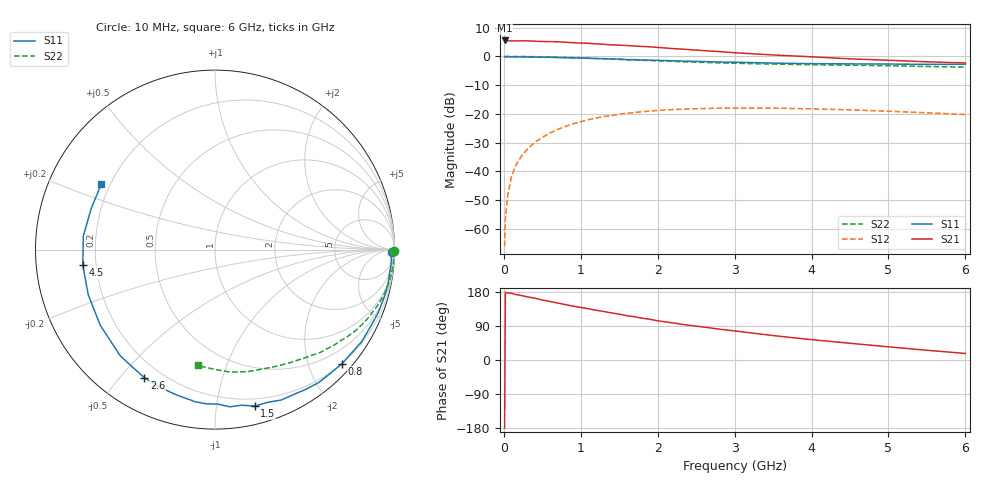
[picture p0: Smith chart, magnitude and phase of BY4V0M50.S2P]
! SIEMENS Small Signal Semiconductors
! BFY420
! Si NPN RF SIEGET Grounded Emitter Transistor in MICRO-X
! VCE = 4 V  IC = 0.5 mA
! Common Emitter S-Parameters:  October  1996
# GHz  S  MA  R  50
!  f  S11  S21  S12  S22
! GHz  MAG  ANG  MAG  ANG  MAG  ANG  MAG  ANG
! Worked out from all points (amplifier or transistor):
!   36 points, 10 MHz to 6 GHz, reference 50 ohm
!   highest |S21| = 5.6 dB at 10 MHz (marker M1)
!   |S21| within 3 dB of that: start of sweep to 2.304 GHz
!   unconditionally stable (mu >= 1): 4.699 GHz to end of sweep
!   at 250 MHz: K = 0.04, MSG = 19.7 dB, |S12| = -34.0 dB
!   at 1.4 GHz: K = 0.16, MSG = 12.3 dB, |S12| = -20.6 dB
!   at 6 GHz: K = 1.46, MAG = 4.9 dB, |S12| = -20.2 dB
!   S11 on the Smith chart (normalised r, x): 10 MHz: 71, -63; 800 MHz: 0.20, -2.59; 1.5 GHz: 0.14, -1.28; 2.6 GHz: 0.14, -0.58; 4.5 GHz: 0.15, -0.06; 6 GHz: 0.17, +0.26
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0.01  0.9843 -0.8  1.896 -179.3  0.0005 88.8  0.9997 -0.3
0.02  0.9772 -1.1  1.896 178.8  0.0015 82.9  0.9999 -0.5
0.05  0.9845 -3.0  1.867 177.2  0.0038 87.3  0.9993 -1.2
0.1  0.9842 -5.4  1.861 176.1  0.0081 86.2  0.996 -2.3
0.15  0.9809 -8.1  1.866 172.8  0.0123 83.4  0.9973 -3.6
0.25  0.9819 -13.4  1.869 169.1  0.02 80.6  0.9958 -5.9
0.4  0.975 -21.1  1.839 163.4  0.0317 76.7  0.9887 -9.5
0.5  0.9667 -26.4  1.817 158.1  0.039 73.6  0.9837 -11.7
0.7  0.9549 -36.9  1.796 150.4  0.0537 67.6  0.9686 -16.3
0.8  0.9509 -42.0  1.768 146.2  0.0607 63.8  0.9601 -18.5
1.1  0.9284 -57.0  1.693 135.1  0.0792 54.9  0.9308 -24.8
1.5  0.8996 -75.7  1.573 121.0  0.0986 43.7  0.8884 -32.4
1.8  0.8605 -89.0  1.491 110.2  0.1092 36.2  0.8565 -37.5
2.2  0.8375 -104.9  1.369 97.8  0.1191 27.0  0.8211 -44.1
2.6  0.815 -118.9  1.261 86.9  0.1239 19.5  0.7861 -49.8
2.8  0.7992 -125.6  1.213 81.4  0.1258 15.9  0.7713 -52.7
3.5  0.7658 -146.6  1.061 64.5  0.1261 5.9  0.7362 -61.8
4  0.7496 -160.5  0.985 53.7  0.1226 0.4  0.7163 -68.3
4.5  0.7416 -173.4  0.908 44.2  0.1177 -4.3  0.7038 -74.9
5  0.7375 174.1  0.857 34.7  0.1113 -6.9  0.689 -82.5
5.5  0.7265 161.5  0.806 25.7  0.1046 -8.3  0.6678 -90.1
6  0.7316 149.9  0.769 17.3  0.0976 -7.8  0.6526 -98.5
